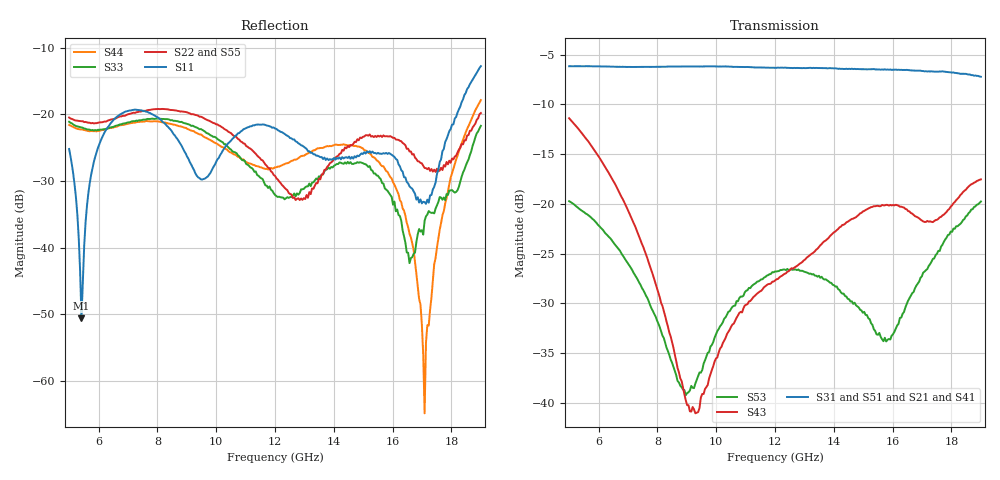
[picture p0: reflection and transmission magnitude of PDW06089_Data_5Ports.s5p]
#	MHz	S	MA	R	50
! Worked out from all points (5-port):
!   301 points, 5 GHz to 19 GHz, reference 50 ohm
!   strongest paths, dB at 5 GHz, 8.5 GHz, 12 GHz, 15.5 GHz, 19 GHz:
!     S31: -6.2, -6.2, -6.3, -6.5, -7.2
!     S51: -6.2, -6.4, -6.6, -6.9, -7.3
!     S21: -6.2, -6.4, -6.6, -6.9, -7.3
!     S41: -6.2, -6.4, -6.6, -6.8, -7.5
!     S43: -11.4, -33.9, -27.7, -20.2, -17.5
!     S53: -19.7, -36.0, -26.8, -33.2, -19.8
!   lowest |S11| = -50.6 dB at 5.42 GHz (marker M1), VSWR 1.01, Z = 50.2 + j0.192 ohm
!   |S11| at or under -10 dB: start of sweep to end of sweep
